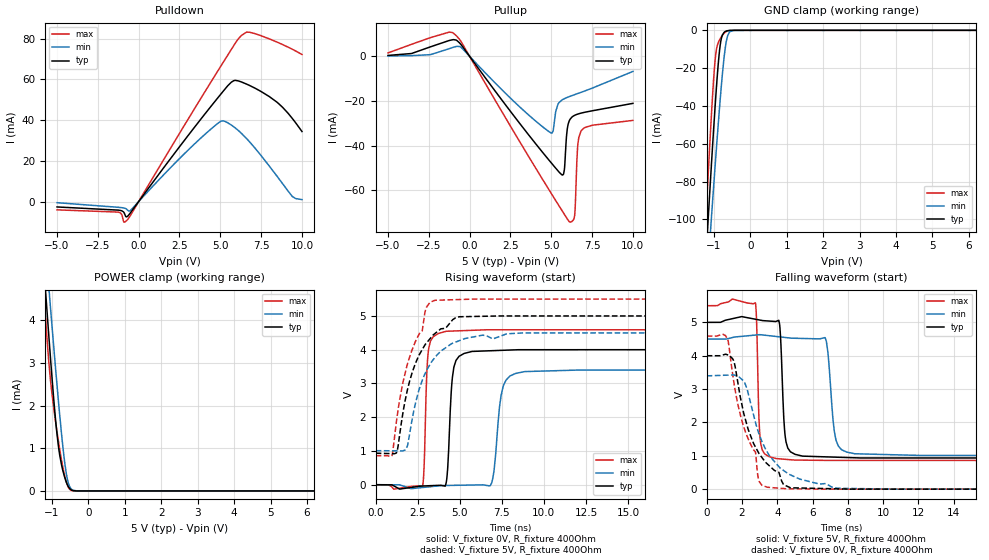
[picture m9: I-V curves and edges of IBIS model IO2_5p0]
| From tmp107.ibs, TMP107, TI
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|   Model
[Model]   IO2_5p0
Model_type   I/O
Polarity   Non-Inverting
Enable   Active-Low
Vinl = 1.5
Vinh = 3.5
Vmeas = 2.5
Vref = 0
Cref = 1pF
Rref = 100000
|   typ   min   max
C_comp   1.060pF   1.035pF   1.082pF
[Voltage Range]   5   4.5   5.5
[Temperature Range]   25   125   -55
[Pullup Reference]   5   4.5   5.5
[Pulldown Reference]   0   -0   0
[Power Clamp Reference]   5   4.5   5.5
[GND Clamp Reference]   0   0   0
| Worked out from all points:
|   slope of the pulldown table from 0 to 0.75 V, typ, clamps not added: 91.8 ohm
|   slope of the pullup table from 0 to 0.75 V, typ, clamps not added: 99.8 ohm
|   GND clamp passes 1 mA (typ) near -0.72 V on its own axis
|   POWER clamp passes 1 mA (typ) near -0.82 V on its own axis
|   falling waveform, V_fixture 5V, R_fixture 400Ohm: 20-80 % time 200ps typ, 325ps min, 143ps max; typ from 5 V to 0.934 V
|   rising waveform, V_fixture 0V, R_fixture 400Ohm: 20-80 % time 253ps typ, 401ps min, 176ps max; typ from 0 V to 4 V
|   rising waveform, V_fixture 5V, R_fixture 400Ohm: 20-80 % time 1.5ns typ, 1.49ns min, 1.56ns max; typ from 0.934 V to 5 V
|   falling waveform, V_fixture 0V, R_fixture 400Ohm: 20-80 % time 1.58ns typ, 1.66ns min, 1.39ns max; typ from 4 V to 0 V
[Pulldown]
|   Voltage   I(typ)   I(min)   I(max)
-5V       -2.65mA    -561.8uA   -4.076mA
-1.25V    -4.21mA    -2.819mA   -5.183mA
-905mV    -5.348mA   -3.176mA   -10.07mA
-740mV    -7.556mA   -3.727mA   -9.359mA
-500mV    -5.463mA   -4.317mA   -6.748mA
3.16V     33.79mA    26.29mA    42.18mA
5.185V    54.24mA    39.59mA    68.45mA
5.83V     59.36mA    36.65mA    76.65mA
6.61V     57.65mA    30.9mA     83.19mA
8.56V     48.15mA    11.5mA     77.97mA
9.415V    40.74mA    2.449mA    74.73mA
10V       34.39mA    941.4uA    72.2mA
[GND Clamp]
|   Voltage   I(typ)   I(min)   I(max)
-5V       -1.451A    -1.265A    -1.626A
-1.25V    -129.7mA   -149.5mA   -110.2mA
-1.145V   -95.07mA   -119.9mA   -71.04mA
-1.07V    -70.99mA   -99.15mA   -44.67mA
-965mV    -39.18mA   -70.82mA   -15.02mA
-920mV    -26.86mA   -59.08mA   -8.877mA
-830mV    -7.975mA   -36.8mA    -4.475mA
-770mV    -2.541mA   -23.43mA   -2.654mA
-665mV    -412.1uA   -6.229mA   -644.7uA
-575mV    -74.11uA   -982.2uA   -97.85uA
-410mV    -1.326uA   -15.73uA   -675.9nA
10V       0A         0A         0A
[Pullup]
|   Voltage   I(typ)   I(min)   I(max)
-5V       414.5uA    192.9uA    1.528mA
-830mV    7.318mA    4.402mA    9.337mA
4.99V     -47.66mA   -34.35mA   -61.33mA
5.41V     -51.3mA    -21.45mA   -66.25mA
5.635V    -53.02mA   -19.66mA   -68.87mA
5.8V      -50.87mA   -18.97mA   -70.78mA
5.98V     -32.47mA   -18.39mA   -72.84mA
6.145V    -28.26mA   -17.92mA   -74.32mA
6.43V     -26.43mA   -17.16mA   -71.37mA
6.61V     -25.9mA    -16.69mA   -40.86mA
6.82V     -25.45mA   -16.14mA   -33.51mA
10V       -21.07mA   -6.747mA   -28.7mA
[POWER Clamp]
|   Voltage   I(typ)   I(min)   I(max)
-5V       53.72mA    48.48mA    61.69mA
-1.235V   5.364mA    6.322mA    4.791mA
-1.16V    4.464mA    5.522mA    3.823mA
-1.07V    3.415mA    4.573mA    2.832mA
-1.01V    2.743mA    3.949mA    2.329mA
-920mV    1.815mA    3.034mA    1.725mA
-800mV    893.7uA    1.873mA    1.03mA
-695mV    447uA      971.9uA    521.7uA
-620mV    232.1uA    468.4uA    244.8uA
-545mV    89.59uA    164.2uA    73.49uA
-470mV    22.46uA    43.78uA    12.19uA
10V       0A         0A         0A
[Ramp]
R_load = 400
|   typ   min   max
dV/dt_r   2.40012/2.4925e-10   2.03803/3.91119e-10   2.75453/1.7548e-10
dV/dt_f   2.43949/1.99226e-10   2.09445/3.21723e-10   2.78371/1.40229e-10
[Falling Waveform]
V_fixture = 5V
V_fixture_min = 4.5V
V_fixture_max = 5.5V
R_fixture = 400Ohm
C_fixture = 0F
|   Time   V(typ)   V(min)   V(max)
0s        5V         4.5V       5.5V
2.757ns   5.095V     4.62V      5.588V
3.057ns   5.065V     4.629V     1.391V
3.941ns   5.032V     4.577V     917.4mV
4.5ns     1.407V     4.544V     893.2mV
5.429ns   991.7mV    4.518V     870.6mV
6.72ns    969mV      4.534V     862.6mV
7.319ns   959.1mV    1.493V     861.4mV
8.392ns   941.2mV    1.062V     861.4mV
50ns      934.2mV    1.009V     860.5mV
[Rising Waveform]
V_fixture = 0V
V_fixture_min = 0V
V_fixture_max = 0V
R_fixture = 400Ohm
C_fixture = 0F
|   Time   V(typ)   V(min)   V(max)
0s        127.5nV    179.5nV    101.4nV
2.768ns   -38.8mV    -83.6mV    -63.19mV
3.152ns   -30.94mV   -64mV      4.042V
4.182ns   49.5mV     -22.61mV   4.545V
4.643ns   3.472V     -18.73mV   4.554V
5.723ns   3.948V     -9.627mV   4.574V
6.895ns   3.97V      57.58mV    4.59V
7.564ns   3.982V     2.891V     4.59V
8.829ns   3.999V     3.349V     4.59V
50ns      4V         3.397V     4.591V
[Rising Waveform]
V_fixture = 5V
V_fixture_min = 4.5V
V_fixture_max = 5.5V
R_fixture = 400Ohm
C_fixture = 0F
|   Time   V(typ)   V(min)   V(max)
0s        934.2mV    1.009V     860.5mV
963.4ps   919.9mV    1.004V     859.7mV
1.274ns   995.2mV    1.003V     2.031V
1.774ns   2.554V     1.031V     3.354V
2.635ns   3.891V     2.908V     4.496V
3.018ns   4.201V     3.377V     5.259V
3.512ns   4.476V     3.765V     5.464V
4.963ns   4.975V     4.266V     5.486V
8.794ns   5V         4.498V     5.499V
50ns      5V         4.5V       5.5V
[Falling Waveform]
|Gnd
V_fixture = 0V
V_fixture_min = 0V
V_fixture_max = 0V
R_fixture = 400Ohm
C_fixture = 0F
|   Time   V(typ)   V(min)   V(max)
0s        4V         3.397V     4.591V
1.183ns   4.027V     3.419V     4.505V
1.563ns   3.791V     3.421V     3.122V
1.958ns   2.627V     3.307V     2.119V
2.757ns   1.27V      2.016V     1.119V
2.976ns   1.058V     1.642V     231.6mV
3.438ns   755.7mV    1.108V     57.94mV
4.744ns   42.43mV    428.6mV    12.24mV
7.399ns   10.01mV    28mV       982.3uV
50ns      304.3nV    424.3nV    228.4nV
